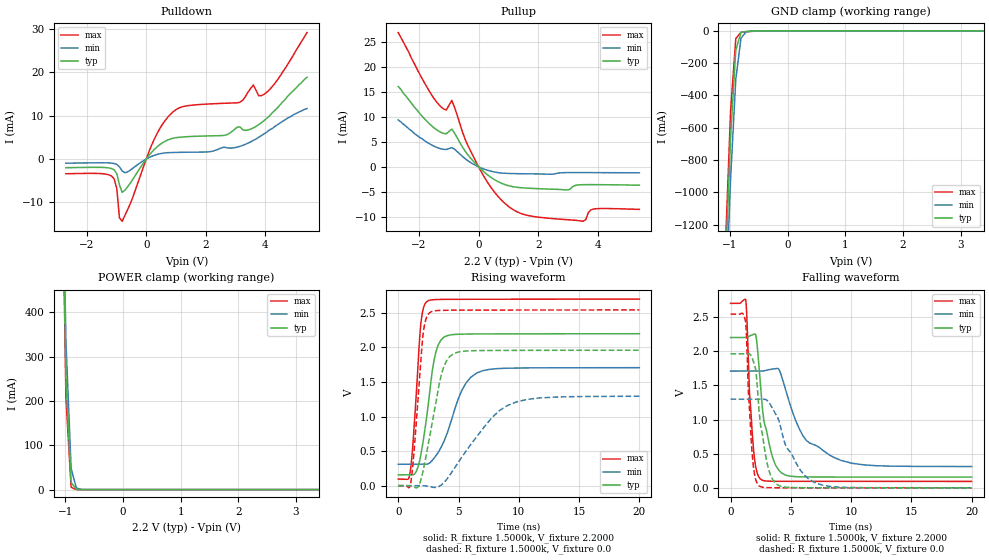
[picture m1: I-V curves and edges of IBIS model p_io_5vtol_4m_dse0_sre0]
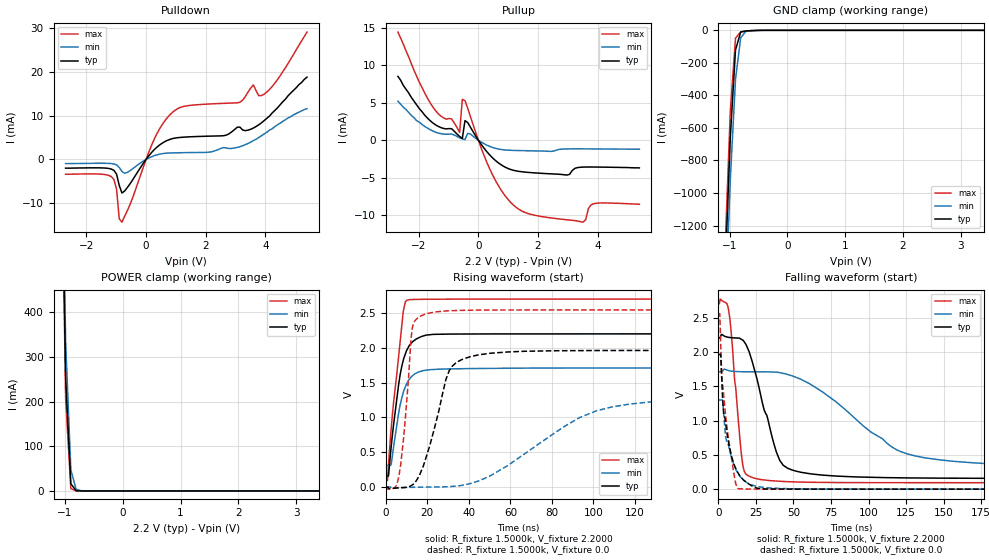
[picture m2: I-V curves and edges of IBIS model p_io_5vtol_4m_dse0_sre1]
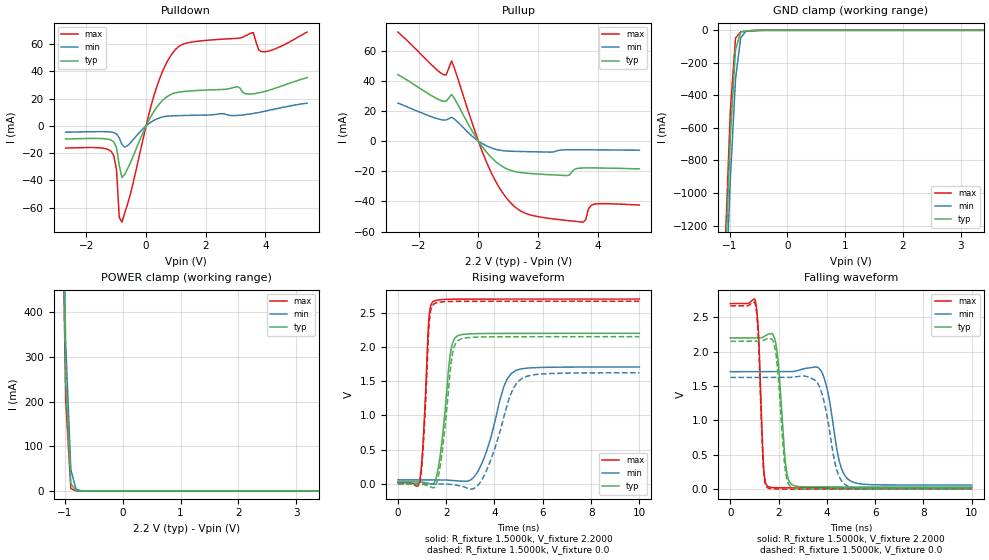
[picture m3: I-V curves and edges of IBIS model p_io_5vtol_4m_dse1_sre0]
| IBIS file nevis_80lqfp_derated.ibs generated by Daphne version: 2018.03.27
[IBIS Ver]   5.0
[Comment Char]   |_char
[File Name]   nevis_80lqfp_derated.ibs
[File Rev]   1
[Date]   Tue Nov  6 17:26:37 2018
[Source]   NXP Viper 2018.03.27
[Notes]
[Disclaimer] IMPORTANT NOTICE
  This information is provided on an AS IS basis and without warranty.
  IN NO EVENT SHALL NXP BE LIABLE FOR INCIDENTAL OR CONSEQUENTIAL
  DAMAGES ARISING FROM USE OF THIS INFORMATION. THIS DISCLAIMER OF
  WARRANTY EXTENDS TO THE USER OF THE INFORMATION, AND TO THEIR CUSTOMERS
  OR USERS OF PRODUCTS  AND IS IN LIEU OF ALL WARRANTIES WHETHER EXPRESS,
  IMPLIED, OR STATUTORY, INCLUDING IMPLIED WARRANTIES OF MERCHANTABILITY
  OR FITNESS FOR PARTICULAR PURPOSE.
  NXP does not represent or warrant that the information furnished
  hereunder is free of infringement of any third party patents,
  copyrights, trade secrets, or other intellectual property rights.
  NXP does not represent or warrant that the information is free of
  defect, or that it meets any particular standard, requirements or need
  of the user of the infomation or their customers.
  NXP reserves the right to change the information in this file
  without notice.
   http://www.nxp.com
[Copyright]   (C) Copyright NXP 2004 - 2018, All Rights Reserved.
|   NEVIS:80LQFP
[Component]   NEVIS:80LQFP
[Manufacturer]   NXP
[Package]
| variable   typ   min   max
R_pkg   0.14792   0.086913   0.16418
L_pkg   3.915e-09   3.208e-09   4.513e-09
C_pkg   6.180e-13   5.453e-13   7.626e-13
[Pin] signal_name   model_name   R_pin   L_pin   C_pin
1   TCK   p_io_5vtol_4m   0.1569   4.463e-09 6.104e-13
2   RESETB   p_vpp_5vtol_4m   0.086913  3.716e-09 7.626e-13
3   GPIOC0   p_io_5vtol_4m   0.1464   4.224e-09 6.498e-13
4   GPIOC1   p_io_5vtol_4m   0.14132   4.089e-09 6.578e-13
5   GPIOC2   p_io_5vtol_4m   0.13836   3.977e-09 6.265e-13
6   GPIOF8   p_io_5vtol_4m   0.13627   3.873e-09 6.056e-13
7   GPIOD6   p_io_5vtol_4m   0.13889   3.853e-09 6.753e-13
8   GPIOD5   p_io_5vtol_4m   0.13733   3.661e-09 5.770e-13
9   GPIOC3   p_io_5vtol_4m   0.13967   3.625e-09 5.687e-13
10   GPIOC4   p_io_5vtol_4m   0.14324   3.260e-09 5.584e-13
11   VSS   GND   NA   NA   NA
12   VDD   POWER   NA   NA   NA
13   GPIOA7   p_io_5vtol_4m   0.14268   3.208e-09 5.596e-13
14   GPIOA6   p_io_5vtol_4m   0.13768   3.627e-09 5.771e-13
15   GPIOA5   p_io_5vtol_4m   0.13834   3.794e-09 6.092e-13
16   GPIOA4   p_io_5vtol_4m   0.14103   3.970e-09 6.163e-13
17   GPIOA0   p_io_5vtol_4m   0.14398   4.103e-09 6.334e-13
18   GPIOA1   p_io_5vtol_4m   0.14886   4.265e-09 6.523e-13
19   GPIOA2   p_io_5vtol_4m   0.15426   4.392e-09 6.811e-13
20   GPIOA3   p_io_5vtol_4m   0.15897   4.513e-09 6.239e-13
21   GPIOB7   p_io_5vtol_4m   0.16119   4.455e-09 6.055e-13
22   GPIOC5   p_io_5vtol_4m   0.089097  3.705e-09 7.594e-13
23   GPIOB6   p_io_5vtol_4m   0.15247   4.133e-09 6.437e-13
24   GPIOB5   p_io_5vtol_4m   0.15127   3.904e-09 6.550e-13
25   GPIOB4   p_io_5vtol_4m   0.15683   3.445e-09 6.248e-13
26   VDDA   POWER   NA   NA   NA
27   VSSA   GND   NA   NA   NA
28   GPIOB0   p_io_5vtol_4m   0.15671   3.227e-09 5.981e-13
29   GPIOB1   p_io_5vtol_4m   0.16081   3.366e-09 5.864e-13
30   VDD   POWER   NA   NA   NA
31   GPIOB2   p_io_5vtol_4m   0.16418   3.339e-09 5.839e-13
32   GPIOA11   p_io_5vtol_4m   0.15928   3.765e-09 5.648e-13
33   GPIOB8   p_io_5vtol_4m   0.15865   3.789e-09 5.728e-13
34   GPIOB3   p_io_5vtol_4m   0.15776   3.412e-09 5.725e-13
35   VDD33   POWER   NA   NA   NA
36   VSS   GND   NA   NA   NA
37   GPIOD7   p_io_5vtol_4m   0.15661   3.718e-09 6.186e-13
38   GPIOG11   p_io_5vtol_4m   0.15508   4.092e-09 6.428e-13
39   GPIOC6   p_io_5vtol_4m   0.15749   4.282e-09 6.708e-13
40   GPIOC7   p_io_5vtol_4m   0.16015   4.420e-09 6.086e-13
41   GPIOC8   p_io_5vtol_4m   0.155   4.392e-09 6.129e-13
42   GPIOC9   p_io_5vtol_4m   0.15023   4.314e-09 6.746e-13
43   GPIOC10   p_io_5vtol_4m   0.14475   4.157e-09 6.325e-13
44   GPIOF0   p_io_5vtol_4m   0.14034   4.038e-09 6.186e-13
45   GPIOF10   p_io_5vtol_4m   0.13729   3.935e-09 5.995e-13
46   GPIOF9   p_io_5vtol_4m   0.13506   3.812e-09 5.800e-13
47   GPIOC11   p_io_5vtol_4m   0.13569   3.773e-09 5.736e-13
48   GPIOC12   p_io_5vtol_4m   0.13431   3.631e-09 5.670e-13
49   GPIOF2   p_io_5vtol_4m   0.13671   3.678e-09 5.521e-13
50   GPIOF3   p_io_5vtol_4m   0.13715   3.575e-09 5.842e-13
51   GPIOF4   p_io_5vtol_4m   0.13922   3.499e-09 5.749e-13
52   GPIOF5   p_io_5vtol_4m   0.14513   3.371e-09 5.453e-13
53   VSS   GND   NA   NA   NA
54   VDD33   POWER   NA   NA   NA
55   GPIOE0   p_io_5vtol_4m   0.14382   3.257e-09 5.801e-13
56   GPIOE1   p_io_5vtol_4m   0.14278   3.728e-09 6.043e-13
57   GPIOG2   p_io_5vtol_4m   0.14594   4.015e-09 5.873e-13
58   GPIOG3   p_io_5vtol_4m   NA   NA   NA
59   GPIOE2   p_io_5vtol_4m   0.15025   4.275e-09 6.580e-13
60   GPIOE3   p_io_5vtol_4m   0.15495   4.361e-09 6.103e-13
61   GPIOC13   p_io_5vtol_4m   0.15782   4.510e-09 6.206e-13
62   GPIOF1   p_io_5vtol_4m   0.15552   4.467e-09 6.836e-13
63   GPIOG0   p_io_5vtol_4m   0.15239   4.349e-09 6.443e-13
64   GPIOG1   p_io_5vtol_4m   0.15   4.246e-09 6.251e-13
65   GPIOE4   p_io_5vtol_4m   0.15123   4.216e-09 6.160e-13
66   GPIOE5   p_io_5vtol_4m   0.14973   4.115e-09 6.183e-13
67   GPIOE6   p_io_5vtol_4m   0.1495   4.063e-09 6.138e-13
68   GPIOE7   p_io_5vtol_4m   0.14975   3.950e-09 6.053e-13
69   GPIOG6   p_io_5vtol_4m   0.15342   4.029e-09 5.810e-13
70   GPIOC14   p_io_5vtol_4m   0.15484   3.948e-09 6.094e-13
71   GPIOC15   p_io_5vtol_4m   0.15791   3.901e-09 6.007e-13
72   GPIOG7   p_io_5vtol_4m   0.16357   3.560e-09 5.812e-13
73   VDD   POWER   NA   NA   NA
74   GPIOF6   p_io_5vtol_4m   0.16081   3.496e-09 6.833e-13
75   GPIOF7   p_io_5vtol_4m   0.16138   3.528e-09 6.113e-13
76   VDD33   POWER   NA   NA   NA
77   VSS   GND   NA   NA   NA
78   TDO   p_io_5vtol_4m   0.16287   3.741e-09 6.499e-13
79   TMS   p_io_5vtol_4m   0.16067   4.282e-09 7.221e-13
80   TDI   p_io_5vtol_4m   0.16215   4.444e-09 6.324e-13
81   NC   NC   NA   NA   NA
[Pin Mapping]   pulldown_ref   pullup_ref
1   NC   NC
2   NC   NC
3   NC   NC
4   NC   NC
5   NC   NC
6   NC   NC
7   NC   NC
8   NC   NC
9   NC   NC
10   NC   NC
11   VSS   NC
12   NC   VDD
13   NC   NC
14   NC   NC
15   NC   NC
16   NC   NC
17   NC   NC
18   NC   NC
19   NC   NC
20   NC   NC
21   NC   NC
22   NC   NC
23   NC   NC
24   NC   NC
25   NC   NC
26   NC   VDDA
27   VSSA   NC
28   NC   NC
29   NC   NC
30   NC   VDD
31   NC   NC
32   NC   NC
33   NC   NC
34   NC   NC
35   NC   VDD33
36   VSS   NC
37   NC   NC
38   NC   NC
39   NC   NC
40   NC   NC
41   NC   NC
42   NC   NC
43   NC   NC
44   NC   NC
45   NC   NC
46   NC   NC
47   NC   NC
48   NC   NC
49   NC   NC
50   NC   NC
51   NC   NC
52   NC   NC
53   VSS   NC
54   NC   VDD33
55   NC   NC
56   NC   NC
57   NC   NC
58   NC   NC
59   NC   NC
60   NC   NC
61   NC   NC
62   NC   NC
63   NC   NC
64   NC   NC
65   NC   NC
66   NC   NC
67   NC   NC
68   NC   NC
69   NC   NC
70   NC   NC
71   NC   NC
72   NC   NC
73   NC   VDD
74   NC   NC
75   NC   NC
76   NC   VDD33
77   VSS   NC
78   NC   NC
79   NC   NC
80   NC   NC
81   NC   NC
|*   Model Selector   *
[Model Selector] p_io_5vtol_4m
p_io_5vtol_4m_dse1_sre0   io, full drive mode without slew rate
p_io_5vtol_4m_dse1_sre1   io, full drive mode with slew rate
p_io_5vtol_4m_dse0_sre0   io, low drive mode without slew rate
p_io_5vtol_4m_dse0_sre1   io, low drive mode with slew rate
| End [Component] NEVIS:80LQFP
| Models and submodels in the file (5): p_io_5vtol_4m_dse0_sre0 (I/O), p_io_5vtol_4m_dse0_sre1 (I/O), p_io_5vtol_4m_dse1_sre0 (I/O), p_io_5vtol_4m_dse1_sre1 (I/O), p_vpp_5vtol_4m (I/O_open_drain)
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[Model] p_io_5vtol_4m_dse0_sre0
|   Model p_io_5vtol_4m_dse0_sre0
| Library cells for typ/min/max conditions are connected as defined below:
|  pad - External Pad
|  ipp_do - Core Input
|  ipp_obe - Output Buffer Enable
|  esd_boost - vdd_s_3v
|  esd_bus - vdd_s_3v
|  ipp_ame - vss_s_lv
|  ipp_dse - vss_s_lv
|  ipp_ina40a_5vtol - NC
|  ipp_ina40b_5vtol - NC
|  ipp_ina_5vtol - NC
|  ipp_ina_mux_3v - NC
|  ipp_ind - NC
|  ipp_ind_3v - NC
|  ipp_pue - vss_s_lv
|  ipp_sre - vss_s_lv
|  tie_3v - vdd_s_3v
|  tie_hi - vdd_s_lv
|  vbuf_3v - vdd_s_3v
|  vdd_bulk_lv - vdd_s_lv
|  vdd_s_3v - vdd_s_3v
|  vdd_s_lv - vdd_s_lv
|  vss_bulk - vss_s_3v
|  vss_s_3v - vss_s_3v
|  vss_s_lv - vss_s_lv
| All other pins connected to ground
Model_type I/O
Polarity   Non-Inverting
Enable   Active-High
Vinl =   0.7700V
Vinh =   1.5400V
Vmeas =  1.1000V
Cref =   25.0000pF
Rref =   1.0000k
Vref =   0.0V
C_comp   2.5897pF   2.5141pF   2.6932pF
[Temperature Range]   25.0000   0.1250k   -40.0000
[Voltage Range]   2.2000V   1.7100V   2.7000V
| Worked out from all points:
|   slope of the pulldown table from 0 to 0.33 V, typ, clamps not added: 128 ohm
|   slope of the pullup table from 0 to 0.33 V, typ, clamps not added: 190 ohm
|   GND clamp passes 1 mA (typ) near -0.56 V on its own axis
|   POWER clamp passes 1 mA (typ) near -0.81 V on its own axis
|   rising waveform, R_fixture 1.5000k, V_fixture 2.2000: 20-80 % time 947ps typ, 1.78ns min, 566ps max; typ from 0.156 V to 2.2 V
|   rising waveform, R_fixture 1.5000k, V_fixture 0.0: 20-80 % time 1.26ns typ, 3.4ns min, 656ps max; typ from 0 V to 1.96 V
|   falling waveform, R_fixture 1.5000k, V_fixture 2.2000: 20-80 % time 953ps typ, 2.78ns min, 464ps max; typ from 2.2 V to 0.158 V
|   falling waveform, R_fixture 1.5000k, V_fixture 0.0: 20-80 % time 819ps typ, 1.91ns min, 430ps max; typ from 1.96 V to 0.001 V
[Pulldown]
|Voltage   I(typ)   I(min)   I(max)
-2.7V     -2mA       -960uA     -3.39mA
-1.17V    -2.19mA    -943uA     -3.913mA
-990mV    -3.359mA   -1.244mA   -6.804mA
-900mV    -5.941mA   -1.821mA   -13.58mA
-810mV    -7.677mA   -2.75mA    -14.34mA
270mV     2.201mA    843.7uA    4.568mA
810mV     4.605mA    1.475mA    10.28mA
3.15V     7.385mA    2.91mA     13.07mA
3.6V      7.17mA     4.3mA      17.03mA
3.78V     7.91mA     5mA        14.56mA
3.96V     8.86mA     5.8mA      14.91mA
5.4V      18.8mA     11.6mA     29.1mA
[Pullup]
|Voltage   I(typ)   I(min)   I(max)
-2.7V     16.1mA     9.4mA      26.9mA
-1.44V    7.55mA     3.98mA     13.23mA
-1.08V    6.637mA    3.488mA    11.41mA
-900mV    7.558mA    3.848mA    13.31mA
-450mV    3.121mA    1.623mA    5.492mA
90mV      -525.5uA   -231.9uA   -998.2uA
540mV     -2.585mA   -1.04mA    -5.11mA
1.08V     -3.888mA   -1.337mA   -8.259mA
2.97V     -4.634mA   -1.154mA   -10.59mA
3.51V     -3.575mA   -1.148mA   -10.91mA
3.87V     -3.565mA   -1.16mA    -8.446mA
5.4V      -3.68mA    -1.2mA     -8.52mA
[GND_clamp]
|Voltage   I(typ)   I(min)   I(max)
-2.7V     -20.35A    -20.38A    -20.37A
-1.08V    -1.486A    -1.737A    -1.339A
-990mV    -654.8mA   -915.7mA   -496.6mA
-900mV    -120.3mA   -300.6mA   -47.98mA
-810mV    -10.43mA   -45.61mA   -9.206mA
-720mV    -3.577mA   -6.172mA   -6.342mA
-540mV    -682.6uA   -563.7uA   -1.265mA
5.4V      0A         0A         0A
[POWER_clamp]
|Voltage   I(typ)   I(min)   I(max)
-2.7V     20.23A     19.96A     20.45A
-1.08V    950.5mA    990.2mA    948mA
-990mV    252.7mA    333.8mA    206.6mA
-900mV    16.05mA    47.59mA    5.278mA
-810mV    508.3uA    3.841mA    61.17uA
-720mV    15.33uA    281.3uA    694.4nA
-630mV    461.8nA    20.43uA    7.955nA
5.4V      0A         0A         0A
[Ramp]
| variable   typ   min   max
dV/dt_r  0.1310/0.6099n   41.9192m/0.9827n   0.3059/0.4620n
dV/dt_f  0.1585/0.2908n   47.3400m/0.4162n   0.3794/0.2202n
R_load = 50.0000
[Rising Waveform]
R_fixture= 1.5000k
V_fixture= 2.2000
V_fixture_min= 1.7100
V_fixture_max= 2.7000
|time   V(typ)   V(min)   V(max)
0s        156.3mV    309.1mV    94.08mV
1.008ns   156.1mV    309mV      214.5mV
1.223ns   156.9mV    309.1mV    604.9mV
1.884ns   453.4mV    309.7mV    2.358V
2.357ns   988.2mV    310.8mV    2.661V
3.11ns    1.925V     428.6mV    2.692V
4.041ns   2.17V      748mV      2.696V
5.622ns   2.194V     1.484V     2.697V
7.005ns   2.196V     1.663V     2.697V
20ns      2.198V     1.707V     2.699V
[Rising Waveform]
R_fixture= 1.5000k
V_fixture= 0.0
V_fixture_min= 0.0
V_fixture_max= 0.0
|time   V(typ)   V(min)   V(max)
0s        2.604nV    511.6nV    74.27pV
1.045ns   -1.902mV   -16.32uV   46.18mV
1.637ns   -19.77mV   562.3uV    1.241V
2.067ns   214.7mV    -137.8uV   2.196V
2.59ns    691.2mV    -13.1mV    2.501V
3.57ns    1.602V     7.719mV    2.537V
4.581ns   1.908V     230.7mV    2.539V
7.764ns   1.956V     982.8mV    2.541V
9.789ns   1.957V     1.211V     2.541V
20ns      1.959V     1.293V     2.542V
[Falling Waveform]
R_fixture= 1.5000k
V_fixture= 2.2000
V_fixture_min= 1.7100
V_fixture_max= 2.7000
|time   V(typ)   V(min)   V(max)
0s        2.2V       1.71V      2.7V
1.266ns   2.199V     1.71V      2.746V
1.857ns   2.244V     1.71V      666.2mV
2.139ns   2.193V     1.71V      267.4mV
2.491ns   1.482V     1.709V     127.5mV
3.471ns   456.6mV    1.739V     97.48mV
4.547ns   189.1mV    1.449V     96.53mV
6.025ns   161.2mV    756.7mV    96.23mV
8.664ns   159.3mV    438.4mV    95.93mV
20ns      158mV      313.1mV    95.07mV
[Falling Waveform]
R_fixture= 1.5000k
V_fixture= 0.0
V_fixture_min= 0.0
V_fixture_max= 0.0
|time   V(typ)   V(min)   V(max)
0s        1.962V     1.3V       2.544V
1.23ns    1.961V     1.299V     2.448V
1.507ns   1.965V     1.299V     1.307V
1.821ns   1.888V     1.299V     441mV
2.08ns    1.736V     1.299V     125.6mV
2.34ns    1.185V     1.299V     33.41mV
3.172ns   261.8mV    1.254V     3.37mV
4.045ns   30.97mV    963.9mV    2.355mV
7.029ns   2.701mV    73.09mV    1.814mV
20ns      1.37mV     2.257mV    877.9uV
[Model] p_io_5vtol_4m_dse0_sre1
|   Model p_io_5vtol_4m_dse0_sre1
| Library cells for typ/min/max conditions are connected as defined below:
|  pad - External Pad
|  ipp_do - Core Input
|  ipp_obe - Output Buffer Enable
|  esd_boost - vdd_s_3v
|  esd_bus - vdd_s_3v
|  ipp_ame - vss_s_lv
|  ipp_dse - vss_s_lv
|  ipp_ina40a_5vtol - NC
|  ipp_ina40b_5vtol - NC
|  ipp_ina_5vtol - NC
|  ipp_ina_mux_3v - NC
|  ipp_ind - NC
|  ipp_ind_3v - NC
|  ipp_pue - vss_s_lv
|  ipp_sre - vdd_s_lv
|  tie_3v - vdd_s_3v
|  tie_hi - vdd_s_lv
|  vbuf_3v - vdd_s_3v
|  vdd_bulk_lv - vdd_s_lv
|  vdd_s_3v - vdd_s_3v
|  vdd_s_lv - vdd_s_lv
|  vss_bulk - vss_s_3v
|  vss_s_3v - vss_s_3v
|  vss_s_lv - vss_s_lv
| All other pins connected to ground
Model_type I/O
Polarity   Non-Inverting
Enable   Active-High
Vinl =   0.7700V
Vinh =   1.5400V
Vmeas =  1.1000V
Cref =   25.0000pF
Rref =   1.0000k
Vref =   0.0V
C_comp   2.5897pF   2.5141pF   2.6932pF
[Temperature Range]   25.0000   0.1250k   -40.0000
[Voltage Range]   2.2000V   1.7100V   2.7000V
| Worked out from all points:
|   slope of the pulldown table from 0 to 0.33 V, typ, clamps not added: 128 ohm
|   slope of the pullup table from 0 to 0.33 V, typ, clamps not added: 190 ohm
|   GND clamp passes 1 mA (typ) near -0.56 V on its own axis
|   POWER clamp passes 1 mA (typ) near -0.81 V on its own axis
|   rising waveform, R_fixture 1.5000k, V_fixture 2.2000: 20-80 % time 5.65ns typ, 5.46ns min, 5.16ns max; typ from 0.156 V to 2.2 V
|   rising waveform, R_fixture 1.5000k, V_fixture 0.0: 20-80 % time 10.2ns typ, 40.8ns min, 4.04ns max; typ from 0 V to 1.96 V
|   falling waveform, R_fixture 1.5000k, V_fixture 2.2000: 20-80 % time 14.9ns typ, 48.1ns min, 5.86ns max; typ from 2.2 V to 0.157 V
|   falling waveform, R_fixture 1.5000k, V_fixture 0.0: 20-80 % time 7.69ns typ, 8.52ns min, 6.7ns max; typ from 1.96 V to 0 V
[Pulldown]
|Voltage   I(typ)   I(min)   I(max)
-2.7V     -2mA       -960uA     -3.39mA
-1.17V    -2.19mA    -943uA     -3.913mA
-990mV    -3.359mA   -1.244mA   -6.804mA
-900mV    -5.941mA   -1.821mA   -13.58mA
-810mV    -7.677mA   -2.75mA    -14.34mA
270mV     2.201mA    843.6uA    4.568mA
810mV     4.605mA    1.475mA    10.28mA
3.15V     7.385mA    2.91mA     13.07mA
3.6V      7.17mA     4.3mA      17.03mA
3.78V     7.91mA     5mA        14.56mA
3.96V     8.86mA     5.8mA      14.91mA
5.4V      18.8mA     11.6mA     29.1mA
[Pullup]
|Voltage   I(typ)   I(min)   I(max)
-2.7V     8.5mA      5.2mA      14.4mA
-1.35V    1.85mA     960uA      3.54mA
-630mV    503.1uA    337.6uA    1.039mA
-540mV    232uA      184.5uA    5.441mA
-450mV    2.62mA     76.25uA    5.267mA
-270mV    1.759mA    833.9uA    3.181mA
450mV     -2.247mA   -924uA     -4.401mA
1.35V     -4.138mA   -1.371mA   -9.168mA
2.97V     -4.634mA   -1.154mA   -10.59mA
3.51V     -3.575mA   -1.148mA   -10.91mA
3.87V     -3.565mA   -1.16mA    -8.446mA
5.4V      -3.68mA    -1.2mA     -8.52mA
[GND_clamp]
|Voltage   I(typ)   I(min)   I(max)
-2.7V     -20.35A    -20.38A    -20.37A
-1.08V    -1.486A    -1.737A    -1.339A
-990mV    -654.8mA   -915.7mA   -496.6mA
-900mV    -120.3mA   -300.6mA   -47.98mA
-810mV    -10.43mA   -45.61mA   -9.206mA
-720mV    -3.577mA   -6.172mA   -6.342mA
-540mV    -682.6uA   -563.7uA   -1.265mA
5.4V      0A         0A         0A
[POWER_clamp]
|Voltage   I(typ)   I(min)   I(max)
-2.7V     20.23A     19.96A     20.45A
-1.08V    950.5mA    990.2mA    948mA
-990mV    252.7mA    333.8mA    206.6mA
-900mV    16.05mA    47.59mA    5.278mA
-810mV    508.3uA    3.841mA    61.17uA
-720mV    15.33uA    281.3uA    694.4nA
-630mV    461.8nA    20.43uA    7.955nA
5.4V      0A         0A         0A
[Ramp]
| variable   typ   min   max
dV/dt_r  0.1311/23.4035n   41.8663m/52.4404n   0.3060/12.8070n
dV/dt_f  0.1582/45.1695n   44.5644m/78.6097n   0.3795/25.2219n
R_load = 50.0000
[Rising Waveform]
R_fixture= 1.5000k
V_fixture= 2.2000
V_fixture_min= 1.7100
V_fixture_max= 2.7000
|time   V(typ)   V(min)   V(max)
0s        156.3mV    309.1mV    94.08mV
815.6ps   157.1mV    309.1mV    105.6mV
1.298ns   167.8mV    309.1mV    331.9mV
2.604ns   593.5mV    333.2mV    856.3mV
6.029ns   1.445V     1.038V     1.844V
7.679ns   1.734V     1.282V     2.341V
8.414ns   1.822V     1.361V     2.529V
10.15ns   1.968V     1.489V     2.684V
22.89ns   2.193V     1.688V     2.698V
250ns     2.2V       1.71V      2.7V
[Rising Waveform]
R_fixture= 1.5000k
V_fixture= 0.0
V_fixture_min= 0.0
V_fixture_max= 0.0
|time   V(typ)   V(min)   V(max)
0s        2.604nV    511.6nV    74.27pV
5.747ns   -13.5mV    -12mV      81.86mV
8.324ns   -9.099mV   -8.182mV   632.2mV
12.6ns    26.88mV    -4.742mV   2.258V
18.59ns   350.7mV    -2.482mV   2.479V
30.52ns   1.672V     3.915mV    2.532V
40.3ns    1.869V     45.21mV    2.54V
93.45ns   1.96V      998.7mV    2.543V
108.8ns   1.961V     1.149V     2.544V
250ns     1.962V     1.298V     2.544V
[Falling Waveform]
R_fixture= 1.5000k
V_fixture= 2.2000
V_fixture_min= 1.7100
V_fixture_max= 2.7000
|time   V(typ)   V(min)   V(max)
0s        2.2V       1.71V      2.7V
6.944ns   2.212V     1.727V     2.608V
8.52ns    2.207V     1.72V      2.32V
15.27ns   2.186V     1.711V     541.7mV
17.35ns   2.146V     1.711V     258.9mV
20.57ns   2.003V     1.71V      188.7mV
38.71ns   541.7mV    1.704V     117.1mV
48.84ns   281.9mV    1.654V     106.5mV
126.3ns   163.9mV    510.7mV    94.31mV
250ns     156.6mV    328.6mV    94.08mV
[Falling Waveform]
R_fixture= 1.5000k
V_fixture= 0.0
V_fixture_min= 0.0
V_fixture_max= 0.0
|time   V(typ)   V(min)   V(max)
0s        1.962V     1.299V     2.544V
1.008ns   1.962V     1.299V     2.55V
1.612ns   1.955V     1.299V     2.128V
2.553ns   1.492V     1.3V       1.576V
3.481ns   1.132V     1.164V     1.404V
4.807ns   982mV      800.2mV    1.092V
8.792ns   484.8mV    465.6mV    459.7mV
12.95ns   246mV      239.2mV    12.26mV
30.99ns   2.45mV     24.33mV    945.8uV
250ns     336.6nV    50.98uV    -9.618nV
[Model] p_io_5vtol_4m_dse1_sre0
|   Model p_io_5vtol_4m_dse1_sre0
| Library cells for typ/min/max conditions are connected as defined below:
|  pad - External Pad
|  ipp_do - Core Input
|  ipp_obe - Output Buffer Enable
|  esd_boost - vdd_s_3v
|  esd_bus - vdd_s_3v
|  ipp_ame - vss_s_lv
|  ipp_dse - vdd_s_lv
|  ipp_ina40a_5vtol - NC
|  ipp_ina40b_5vtol - NC
|  ipp_ina_5vtol - NC
|  ipp_ina_mux_3v - NC
|  ipp_ind - NC
|  ipp_ind_3v - NC
|  ipp_pue - vss_s_lv
|  ipp_sre - vss_s_lv
|  tie_3v - vdd_s_3v
|  tie_hi - vdd_s_lv
|  vbuf_3v - vdd_s_3v
|  vdd_bulk_lv - vdd_s_lv
|  vdd_s_3v - vdd_s_3v
|  vdd_s_lv - vdd_s_lv
|  vss_bulk - vss_s_3v
|  vss_s_3v - vss_s_3v
|  vss_s_lv - vss_s_lv
| All other pins connected to ground
Model_type I/O
Polarity   Non-Inverting
Enable   Active-High
Vinl =   0.7700V
Vinh =   1.5400V
Vmeas =  1.1000V
Cref =   25.0000pF
Rref =   1.0000k
Vref =   0.0V
C_comp   2.5897pF   2.5141pF   2.6932pF
[Temperature Range]   25.0000   0.1250k   -40.0000
[Voltage Range]   2.2000V   1.7100V   2.7000V
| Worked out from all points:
|   slope of the pulldown table from 0 to 0.33 V, typ, clamps not added: 25.7 ohm
|   slope of the pullup table from 0 to 0.33 V, typ, clamps not added: 38.3 ohm
|   GND clamp passes 1 mA (typ) near -0.56 V on its own axis
|   POWER clamp passes 1 mA (typ) near -0.81 V on its own axis
|   rising waveform, R_fixture 1.5000k, V_fixture 2.2000: 20-80 % time 357ps typ, 774ps min, 207ps max; typ from 0.031 V to 2.2 V
|   rising waveform, R_fixture 1.5000k, V_fixture 0.0: 20-80 % time 368ps typ, 842ps min, 213ps max; typ from 0 V to 2.15 V
|   falling waveform, R_fixture 1.5000k, V_fixture 2.2000: 20-80 % time 259ps typ, 472ps min, 164ps max; typ from 2.2 V to 0.032 V
|   falling waveform, R_fixture 1.5000k, V_fixture 0.0: 20-80 % time 266ps typ, 512ps min, 164ps max; typ from 2.15 V to 0.001 V
[Pulldown]
|Voltage   I(typ)   I(min)   I(max)
-2.7V     -9.58mA    -4.57mA    -16.24mA
-1.17V    -10.45mA   -4.486mA   -18.73mA
-990mV    -15.98mA   -5.899mA   -32.6mA
-900mV    -28.96mA   -8.728mA   -67.1mA
-810mV    -37.86mA   -13.49mA   -70.68mA
270mV     10.92mA    4.187mA    22.64mA
990mV     24.34mA    7.491mA    56.19mA
3.06V     28.9mA     7.71mA     64.33mA
3.6V      23.63mA    9.2mA      68.56mA
3.78V     24.28mA    9.8mA      55.81mA
4.05V     25.71mA    11.1mA     54.67mA
5.4V      35.5mA     16.7mA     68.9mA
[Pullup]
|Voltage   I(typ)   I(min)   I(max)
-2.7V     44mA       25.2mA     72.2mA
-1.17V    26.34mA    13.97mA    43.99mA
-1.08V    26.42mA    14.03mA    43.92mA
-900mV    30.88mA    15.71mA    53mA
360mV     -9.303mA   -3.93mA    -17.88mA
810mV     -16.87mA   -6.301mA   -34.14mA
1.35V     -20.64mA   -6.862mA   -45.44mA
2.97V     -22.84mA   -5.752mA   -52.58mA
3.51V     -17.79mA   -5.736mA   -53.71mA
3.69V     -17.74mA   -5.75mA    -45.02mA
3.87V     -17.76mA   -5.78mA    -41.87mA
5.4V      -18.37mA   -6.03mA    -42.34mA
[GND_clamp]
|Voltage   I(typ)   I(min)   I(max)
-2.7V     -20.35A    -20.38A    -20.37A
-1.08V    -1.486A    -1.737A    -1.339A
-990mV    -654.8mA   -915.7mA   -496.6mA
-900mV    -120.3mA   -300.6mA   -47.98mA
-810mV    -10.43mA   -45.61mA   -9.206mA
-720mV    -3.577mA   -6.172mA   -6.342mA
-540mV    -682.6uA   -563.7uA   -1.265mA
5.4V      0A         0A         0A
[POWER_clamp]
|Voltage   I(typ)   I(min)   I(max)
-2.7V     20.23A     19.96A     20.45A
-1.08V    950.5mA    990.2mA    948mA
-990mV    252.7mA    333.8mA    206.6mA
-900mV    16.05mA    47.59mA    5.278mA
-810mV    508.3uA    3.841mA    61.17uA
-720mV    15.33uA    281.3uA    694.4nA
-630mV    461.8nA    20.43uA    7.955nA
5.4V      0A         0A         0A
[Ramp]
| variable   typ   min   max
dV/dt_r  0.6013/0.6303n   0.2061/1.0273n   1.0878/0.3490n
dV/dt_f  0.7290/0.3945n   0.2308/0.5522n   1.2634/0.2266n
R_load = 50.0000
[Rising Waveform]
R_fixture= 1.5000k
V_fixture= 2.2000
V_fixture_min= 1.7100
V_fixture_max= 2.7000
|time   V(typ)   V(min)   V(max)
0s        31.17mV    60.02mV    18.84mV
919.5ps   30.78mV    60.01mV    91.53mV
1.282ns   8.226mV    60.09mV    2.413V
1.447ns   3.959mV    60.27mV    2.659V
1.758ns   435.1mV    60.48mV    2.69V
2.169ns   1.9V       54.09mV    2.697V
2.459ns   2.16V      45.47mV    2.698V
3.365ns   2.196V     217.8mV    2.699V
4.869ns   2.199V     1.655V     2.699V
10ns      2.199V     1.708V     2.7V
[Rising Waveform]
R_fixture= 1.5000k
V_fixture= 0.0
V_fixture_min= 0.0
V_fixture_max= 0.0
|time   V(typ)   V(min)   V(max)
0s        554.5pV    116.8nV    15.42pV
925ps     -422.4uV   -11.58uV   53.71mV
1.296ns   -31.52mV   76.09uV    2.353V
1.461ns   -54.01mV   295.3uV    2.619V
1.698ns   153.9mV    642.5uV    2.652V
2.196ns   1.759V     -7.306mV   2.665V
2.486ns   2.094V     -20.73mV   2.666V
3.477ns   2.147V     59.83mV    2.667V
5.162ns   2.15V      1.547V     2.667V
10ns      2.151V     1.624V     2.667V
[Falling Waveform]
R_fixture= 1.5000k
V_fixture= 2.2000
V_fixture_min= 1.7100
V_fixture_max= 2.7000
|time   V(typ)   V(min)   V(max)
0s        2.2V       1.71V      2.7V
1.054ns   2.2V       1.71V      2.712V
1.378ns   2.215V     1.71V      342.1mV
1.534ns   2.249V     1.71V      48.36mV
1.907ns   2.075V     1.71V      21.05mV
2.282ns   395.9mV    1.709V     19.8mV
2.523ns   76.4mV     1.711V     19.62mV
3.755ns   32.34mV    1.726V     19.35mV
4.981ns   31.9mV     120.2mV    19.29mV
10ns      31.69mV    61.08mV    19.18mV
[Falling Waveform]
R_fixture= 1.5000k
V_fixture= 0.0
V_fixture_min= 0.0
V_fixture_max= 0.0
|time   V(typ)   V(min)   V(max)
0s        2.151V     1.626V     2.668V
1.036ns   2.151V     1.626V     2.693V
1.371ns   2.165V     1.626V     306.7mV
1.533ns   2.192V     1.626V     23.56mV
1.871ns   2.021V     1.626V     2.171mV
2.263ns   324.8mV    1.626V     928.9uV
2.513ns   34.93mV    1.627V     748.9uV
3.68ns    1.097mV    1.504V     496.2uV
4.791ns   728.7uV    59.37mV    439.6uV
10ns      501.2uV    942.9uV    324.1uV
